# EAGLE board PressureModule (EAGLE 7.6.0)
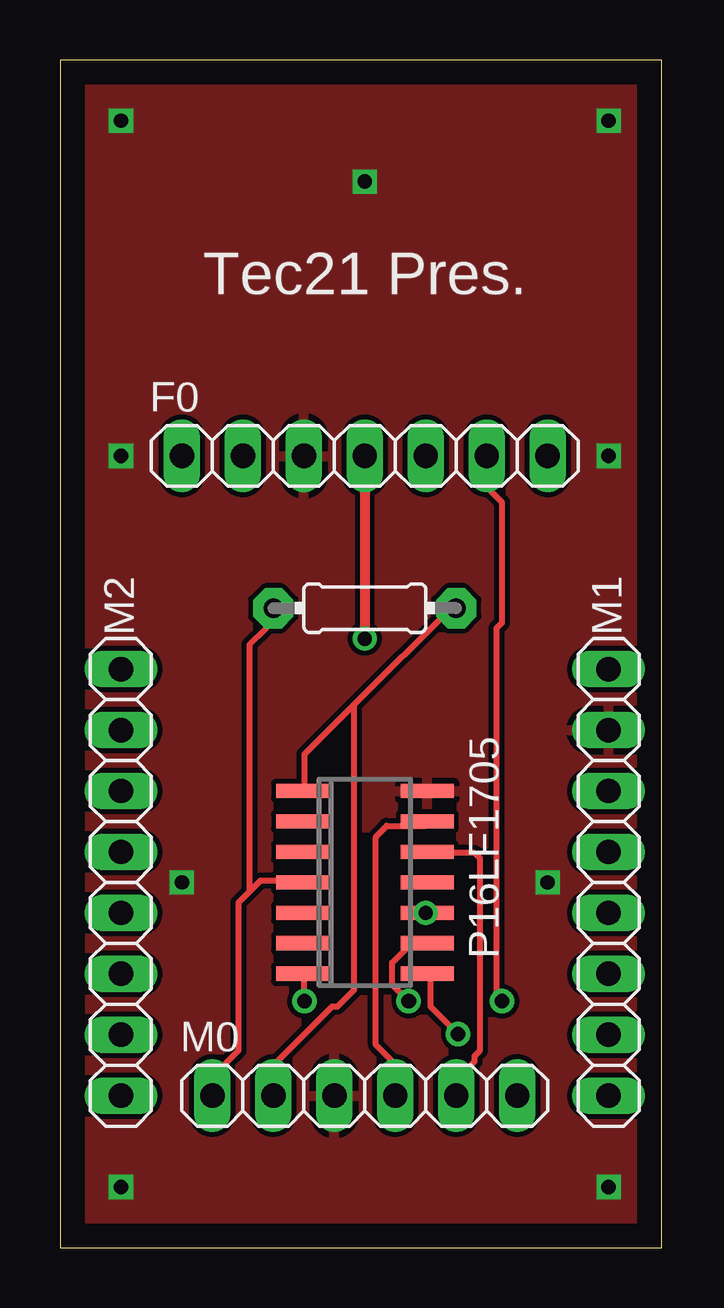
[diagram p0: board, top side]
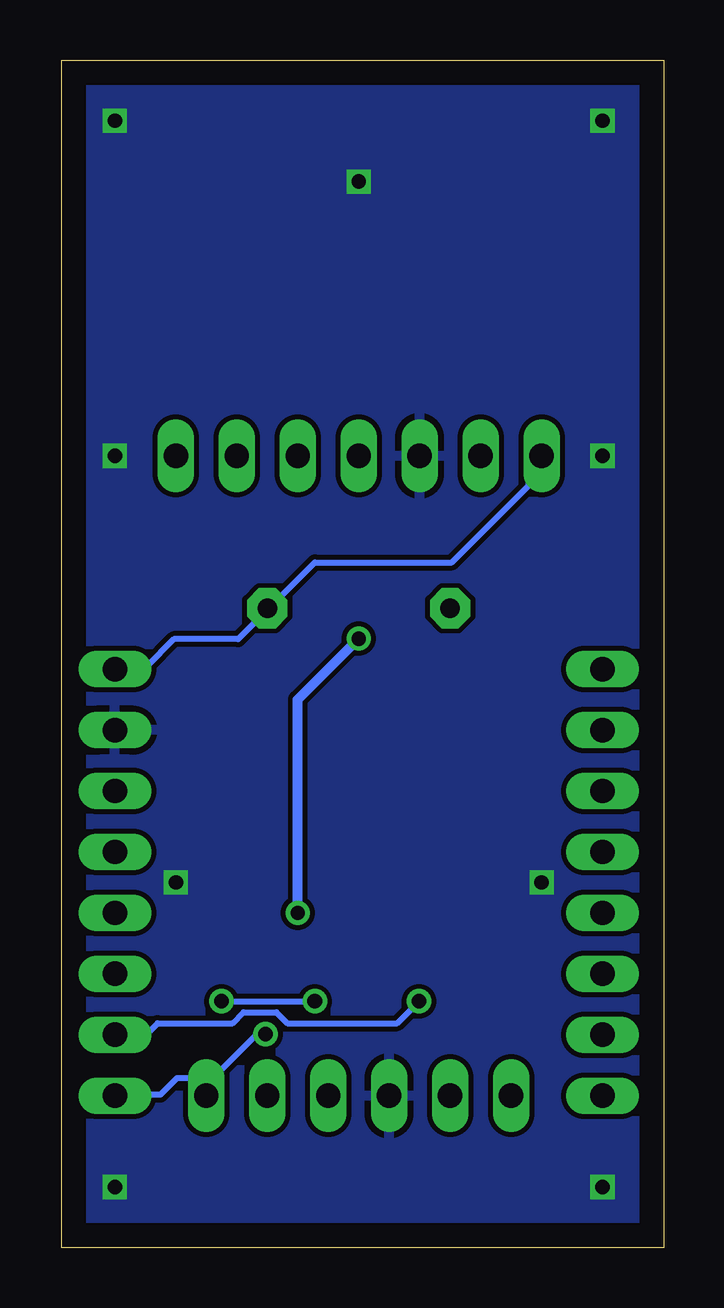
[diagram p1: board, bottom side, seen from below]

Size 25.07 x 49.52 mm. Coordinates in mm from the lower left corner, seen from the top.
Outline: 0,0 25.07,0 25.07,49.52 0,49.52 0,0
Copper layers (1*16): Top 0.035mm / dielectric 1.5mm / Bottom 0.035mm
Design rules "default": minimum track width 10mil, minimum drill 24mil, track to track 8mil, track to pad 8mil, pad to pad 8mil, via to via 8mil, smd to smd 8mil, copper to edge 40mil, drill to drill 8mil, minimum pad ring 10mil, minimum via ring 8mil, stop-mask expansion 4mil, vias tented up to drill 0mil, thermal gap 10mil

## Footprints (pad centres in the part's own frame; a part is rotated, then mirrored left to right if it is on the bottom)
0204/7 = drill 0.813 pad 1.676 octagon: 1 -3.81,0; 2 3.81,0
1X07 = drill 1.016 long: 1 -7.62,0; 2 -5.08,0; 3 -2.54,0; 4 0,0; 5 2.54,0; 6 5.08,0; 7 7.62,0
1X06 = drill 1.016 long: 1 -6.35,0; 2 -3.81,0; 3 -1.27,0; 4 1.27,0; 5 3.81,0; 6 6.35,0
1X08 = drill 1.016 long: 1 -8.89,0; 2 -6.35,0; 3 -3.81,0; 4 -1.27,0; 5 1.27,0; 6 3.81,0; 7 6.35,0; 8 8.89,0
SO-14 = smd 0.6 x 2.2: 1 -3.81,-2.6; 2 -2.54,-2.6; 3 -1.27,-2.6; 4 0,-2.6; 5 1.27,-2.6; 6 2.54,-2.6; 7 3.81,-2.6; 8 3.81,2.6; 9 2.54,2.6; 10 1.27,2.6; 11 0,2.6; 12 -1.27,2.6; 13 -2.54,2.6; 14 -3.81,2.6

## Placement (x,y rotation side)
10K  10k  [0204/7]  12.7,26.67 0 top
F0  [1X07]  12.7,33.02 0 top
M0  [1X06]  12.7,6.35 0 top
M1  [1X08]  22.86,15.24 270 top
M2  [1X08]  2.54,15.24 270 top
P16LF1705  PIC16F676SL  [SO-14]  12.7,15.24 270 top

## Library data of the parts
10K = adafruit
F0 M0 M1 M2 = pinhead
P16LF1705 = microchip; MF: MICROCHIP; MPN: PIC16F676-I/SL; OC_FARNELL: 9760520; OC_NEWARK: 92C4557

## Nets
CCL: M1.7 P16LF1705.7
CDA: M1.8 P16LF1705.8
GND: F0.3 M0.3 M1.2 P16LF1705.14
LCL: F0.6 P16LF1705.9
LDA: F0.4 P16LF1705.10
MCLR: 10K.1 M0.1 P16LF1705.4
N$8: F0.2
PGC: M0.5 P16LF1705.12
PGD: M0.4 P16LF1705.13
VDD: 10K.2 F0.1 M0.2 M1.1 P16LF1705.1

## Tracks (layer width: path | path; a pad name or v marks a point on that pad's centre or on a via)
CCL  (via drill 0.61)
  Top 0.254: v10.18,10.29 10.18,11.43 P16LF1705.7
  Bottom 0.254: v10.18,10.29 11.1,9.37 15.67,9.37 16.13,9.83 17.5,9.83 17.96,9.37 21.08,9.37 21.54,8.91 22.68,8.91 M1.7
CDA  (via drill 0.61)
  Top 0.254: v16.59,8.91 15.44,10.06 15.44,11.43 P16LF1705.8
  Bottom 0.254: v16.59,8.91 16.94,8.91 18.77,7.09 20.27,7.09 20.95,6.4 21.41,6.4 M1.8
GND  (via drill 0.6)
  other vias: 2.54,46.99 22.86,46.99 22.86,33.02 2.54,33.02 12.7,44.45 5.08,15.24 20.32,15.24 2.54,2.54 22.86,2.54
  pour Top: -1.27,50.8 26.67,50.8 26.67,-1.27 -1.27,-1.27
  pour Bottom: -1.27,50.8 26.67,50.8 26.67,-1.27 -1.27,-1.27
LCL  (via drill 0.61)
  Top 0.254: v14.53,10.29 13.84,10.97 13.84,11.89 14.53,12.57 15.21,12.57 P16LF1705.9 | v18.41,10.29 18.19,10.52 18.19,25.83 18.41,26.06 18.41,31.09 17.96,31.55 17.96,32.92 F0.6
  Bottom 0.254: v18.41,10.29 v14.53,10.29
LDA  (via drill 0.6)
  Top 0.254: P16LF1705.10 15.44,13.95 v15.24,13.97
  Top 0.406: F0.4 v12.7,25.4
  Bottom 0.406: v15.24,13.97 15.24,22.86 v12.7,25.4
MCLR
  Top 0.254: 7.9,14.86 7.44,14.4 7.44,8.23 6.53,7.32 6.53,6.4 M0.1 | 7.9,14.86 8.36,15.32 9.96,15.32 P16LF1705.4 | 7.9,14.86 7.9,25.15 8.59,25.83 8.59,26.29 8.81,26.52 10K.1
PGC
  Top 0.254: P16LF1705.12 15.44,16.46 17.27,16.46 17.5,16.23 17.5,8.23 17.27,8 17.27,7.77 16.59,7.09 16.59,6.4 M0.5
PGD
  Top 0.254: P16LF1705.13 15.21,17.6 13.61,17.6 13.16,17.14 13.16,8.46 14.07,7.54 14.07,6.4 M0.4
VDD
  Top 0.254: 12.24,22.63 16.36,26.75 10K.2 | 12.24,22.63 10.18,20.57 10.18,19.2 P16LF1705.1 | 12.24,22.63 12.24,10.74 11.56,10.06 11.33,10.06 9.04,7.77 9.04,6.4 M0.2
  Bottom 0.254: F0.1 5.16,32.92 5.61,32.46 5.61,31.77 8.81,28.57 14.53,28.57 16.36,26.75 10K.2 16.59,26.52 17.73,25.38 20.4,25.38 21.54,24.23 22.68,24.23 M1.1

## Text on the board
tPlace: Tec21 Pres.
